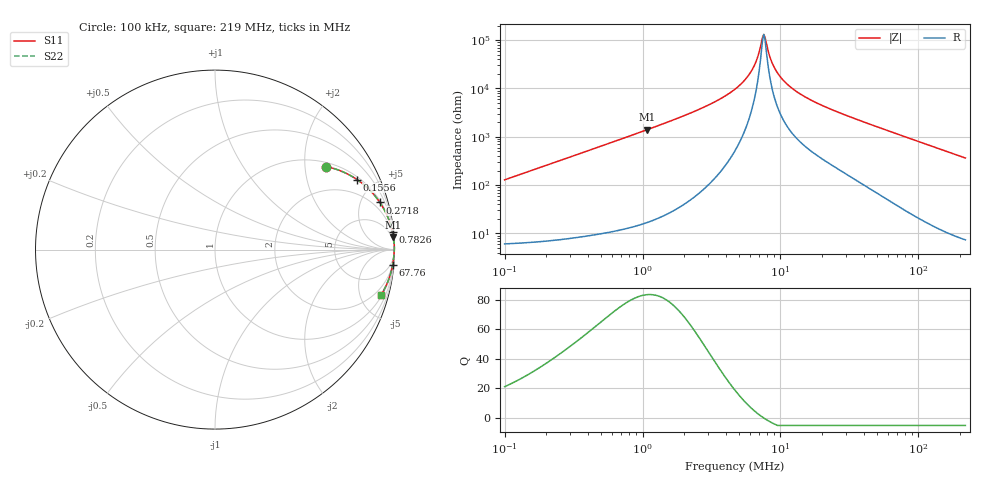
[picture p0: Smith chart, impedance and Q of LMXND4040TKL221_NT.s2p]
! LMXND4040TKL221_NT  S-PARAMETER MODEL  ( Standard Model )
! Model Generated by TAIYO YUDEN Corporation (https://www.yuden.co.jp/en/)
! Version 1.0
! TAIYO YUDEN Control No. 20250409
! Copyright(c) 2025 TAIYO YUDEN CO.,LTD. All Rights Reserved.
! Product Description (link to TY-COMPAS)
! https://ds.yuden.co.jp/TYCOMPAS/or/detail?pn=LMXND4040TKL221MNT&u=M
! Products Name : Inductors
! Characteristics :
!  Inductance : 220 [uH] , SRF(min) : 4.0 [MHz] , DC Resistance(max) : 4.56 [Ohm]
!  Rated Current : Saturation  275 [mA] , Temp Rise  280 [mA] (40 [degC])
!  Case Size : 4.0 x 4.0 / 0.157 x 0.157 [mm/inch] , Thickness : 1.8 / 0.071 [mm/inch]
!  (Conditions: Temperature = 25 [degC] , DC Bias Current = 0 [A])
! External Node Assignments :
!  1  o---GGG---o  2
! GND o---------o GND
! Frequency Range : 0.1MHz  -  218.972167MHz  [ 402 STEP ]
# MHz S RI R 50
! Freq[MHz].  S11 Real  S11 Imag  S21 Real  S21 Imag  S12 Real  S12 Imag  S22 Real  S22 Imag
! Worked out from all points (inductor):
!   401 points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, 100 kHz to 219 MHz, reference 50 ohm
!   read as one part in series: L = 204 uH near 103.9 kHz
!   highest Q = 83.3 at 1.085 MHz (marker M1), where L = 207 uH
!   self-resonance near 7.568 MHz
!   S11 on the Smith chart (normalised r, x): 100 kHz: 1.12, +2.57; 155.6 kHz: 1.13, +3.99; 271.8 kHz: 1.15, +6.96; 782.6 kHz: 1, +20; 67.76 MHz: 2, -24; 219 MHz: 1.15, -7.28
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0.1  0.6179 0.4628  0.3821 -0.4628  0.3821 -0.4628  0.6179 0.4628
0.155622  0.7917 0.3901  0.2083 -0.3901  0.2083 -0.3901  0.7917 0.3901
0.271801  0.9188 0.2624  0.0812 -0.2624  0.0812 -0.2624  0.9188 0.2624
0.362673  0.9522 0.2044  0.0478 -0.2044  0.0478 -0.2044  0.9522 0.2044
0.782626  0.989 0.0981  0.011 -0.0981  0.011 -0.0981  0.989 0.0981
1.085227  0.9942 0.0705  0.00585 -0.0705  0.00585 -0.0705  0.9942 0.0705
1.315317  0.996 0.0577  0.00405 -0.0577  0.00405 -0.0577  0.996 0.0577
3.006922  0.999 0.022  0.000975 -0.022  0.000975 -0.022  0.999 0.022
4.770297  0.9993 0.00988  0.000654 -0.00988  0.000654 -0.00988  0.9993 0.00988
5.563566  0.9994 0.00645  0.000648 -0.00645  0.000648 -0.00645  0.9994 0.00645
6.243945  0.9993 0.00399  0.000672 -0.00399  0.000672 -0.00399  0.9993 0.00399
6.743152  0.9993 0.00239  0.0007 -0.00239  0.0007 -0.00239  0.9993 0.00239
7.282271  0.9993 0.000806  0.000739 -0.000806  0.000739 -0.000806  0.9993 0.000806
7.567785  0.9992 1.86e-05  0.000763 -1.86e-05  0.000763 -1.86e-05  0.9992 1.86e-05
7.864493  0.9992 -0.000767  0.000789 0.000767  0.000789 0.000767  0.9992 -0.000767
8.826256  0.9991 -0.00313  0.000883 0.00313  0.000883 0.00313  0.9991 -0.00313
9.905636  0.999 -0.00551  0.001 0.00551  0.001 0.00551  0.999 -0.00551
12.23892  0.9987 -0.01  0.00128 0.01  0.00128 0.01  0.9987 -0.01
16.97108  0.9981 -0.0178  0.00187 0.0178  0.00187 0.0178  0.9981 -0.0178
61.54953  0.9915 -0.0757  0.00854 0.0757  0.00854 0.0757  0.9915 -0.0757
67.76097  0.9901 -0.0834  0.00986 0.0834  0.00986 0.0834  0.9901 -0.0834
218.9722  0.9254 -0.2528  0.0746 0.2528  0.0746 0.2528  0.9254 -0.2528
